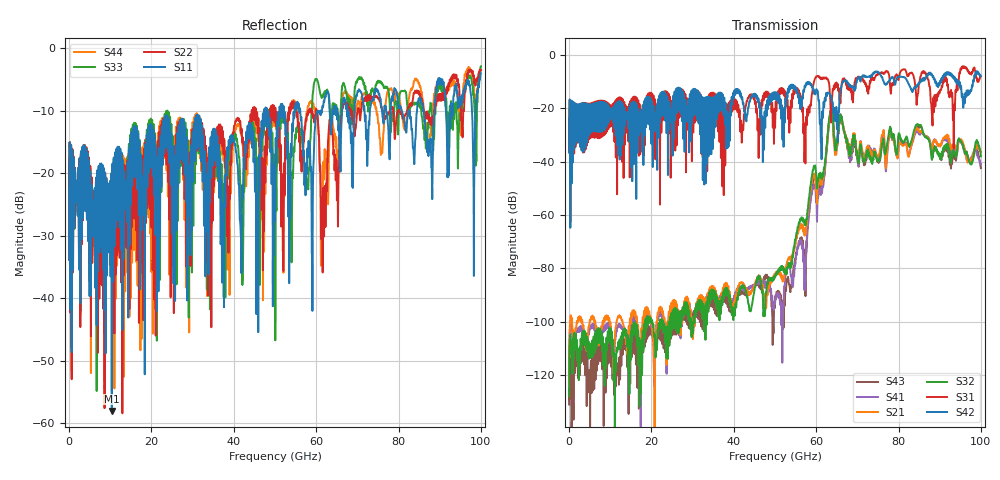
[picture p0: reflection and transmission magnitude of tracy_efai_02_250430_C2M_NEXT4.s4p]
!! PART DESCRIPTION: TE 224G+ VSR Channel- Chip to module, IO connector to CPC(Co-packaged connector) through over the board cable
!! CHANNEL DESCRIPTION: Module trace -> Mated IO 224G+ Connector -> Internal Cable Termination -> 30AWG 300mm Cable -> Cable
!!  termination + CPC connector(No footprint or package included)
!! MODEL REVISION:  Rev 3, Created on April 25, 2025
!! MODEL STATUS: Development
!! MODEL GEOMETRY: 8 Pair Channel
!! MODEL FREQUENCY RANGE: 0 GHz to 100 GHz in 10.00 MHz frequency steps
!! MODEL EDGE RATE LIMITATION: 5ps (Using conservative 0.5/Fmax rule of thumb)
!! PORT DEFINITIONS:
!! Port  1  ----->  Module Side  -->  Host Side, A Row  <-----  Port  2
!! Port  3  ----->  Module Side  -->  Host Side, A Row  <-----  Port  4
# GHz S MA R 45
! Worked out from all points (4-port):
!   10000 points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, 10 MHz to 100 GHz, reference 45 ohm
!   strongest paths, dB at 10 MHz, 25.01 GHz, 50.01 GHz, 75.01 GHz, 100 GHz:
!     S42: -36.5, -18.1, -14.5, -6.3, -8.0
!     S31: -36.5, -27.8, -27.1, -7.4, -8.0
!     S32: -127.8, -103.1, -83.4, -39.5, -38.0
!     S21: -124.3, -95.4, -82.5, -38.1, -36.5
!     S41: -125.5, -97.2, -93.0, -38.8, -40.8
!     S43: -130.9, -105.1, -92.1, -40.2, -42.4
!   lowest |S11| = -58.0 dB at 10.38 GHz (marker M1), VSWR 1.00, Z = 45 + j0.107 ohm
!   |S11| at or under -10 dB: start of sweep to 47.36 GHz; 48.09 GHz to 51.06 GHz (2.963 GHz wide, 5.98 % of centre); 56.14 GHz to 60.39 GHz (4.253 GHz wide, 7.3 % of centre)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
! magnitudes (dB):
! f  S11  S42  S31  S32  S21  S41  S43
! 10 MHz  -33.8  -36.5  -36.5  -127.8  -124.3  -125.5  -130.9
! 10.38 GHz  -58.0  -22.4  -23.2  -103.7  -104.4  -104.5  -107.6
! 51.98 GHz  -10.4  -21.7  -13.9  -79.8  -83.4  -93.9  -94.5
! 54.18 GHz  -12.1  -11.3  -14.8  -76.1  -75.1  -84.9  -82.7
! 57.36 GHz  -21.4  -12.1  -36.2  -62.6  -65.5  -78.8  -86.7
! 63.61 GHz  -13.7  -15.5  -24.3  -21.1  -22.2  -22.2  -21.0
! 100 GHz  -4.0  -8.0  -8.0  -38.0  -36.5  -40.8  -42.4
